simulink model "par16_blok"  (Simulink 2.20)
settings: Solver=ode45  StartTime=0.0  StopTime=320.0  MaxStep=0.01  RelTol=1e-3  AbsTol=1e-6
libraries: simulink x2

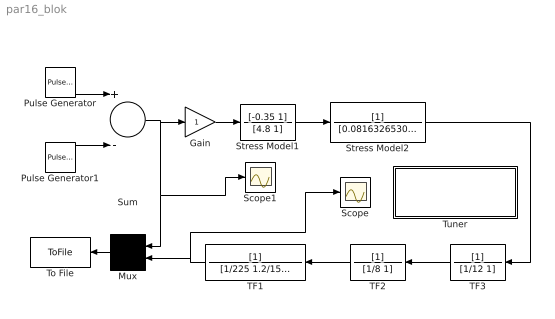
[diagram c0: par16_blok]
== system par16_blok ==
  Gain : Gain  Gain=1
  Mux : Mux  Orientation=left  Inputs=2
  Pulse Generator : simulink/Sources/Pulse Generator  period=40  duty=50  amplitude=1  start=0
  Pulse Generator1 : simulink/Sources/Pulse Generator  period=40  duty=50  amplitude=1  start=20
  Scope : Scope
  Scope1 : Scope
  Stress Model1 : TransferFcn  Numerator=[-0.35 1]  Denominator=[4.8 1]
  Stress Model2 : TransferFcn  Numerator=[1]  Denominator=[0.0816326530612245 0.114285714285714 1]
  Sum : Sum  Inputs=+-
  TF1 : TransferFcn  Orientation=left  Numerator=[1]  Denominator=[1/225 1.2/15 1]
  TF2 : TransferFcn  Orientation=left  Numerator=[1]  Denominator=[1/8 1]
  TF3 : TransferFcn  Orientation=left  Numerator=[1]  Denominator=[1/12 1]
  To File : ToFile  Orientation=left  Filename=bmd16.mat  MatrixName=mbio  SampleTime=0.01
  Tuner : Subsystem  mask(Stress Level 1){name1='par16_blok/Stress Model1', name2='par16_blok/Stress Model2', fname='par16'}
      mask prompts: name1 "'Block Name 1' :"; name2 "'Block Name 2 ' :"; fname "'FileName' :"
      mask init:
      | name1=@1; name2=@2; fname=@3;
      | efname=[fname '.dat'];         eval(['load ' efname]);
      | par=eval(fname);    lp=length(par(1,:));
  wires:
  Gain/1 -> Stress Model1/1
  Stress Model1/1 -> Stress Model2/1
  Stress Model2/1 -> TF3/1
  TF3/1 -> TF2/1
  TF2/1 -> TF1/1
  Mux/1 -> To File/1
  Sum/1 -> Gain/1, Mux/1, Scope1/1
  Pulse Generator1/1 -> Sum/2
  Pulse Generator/1 -> Sum/1
  TF1/1 -> Mux/2, Scope/1

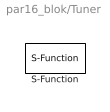
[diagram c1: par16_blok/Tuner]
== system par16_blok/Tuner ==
  S-Function : S-Function  FunctionName=S_bm5_sl  Parameters=name1,name2,par,lp  PortCounts=[]  SFunctionModules=''
